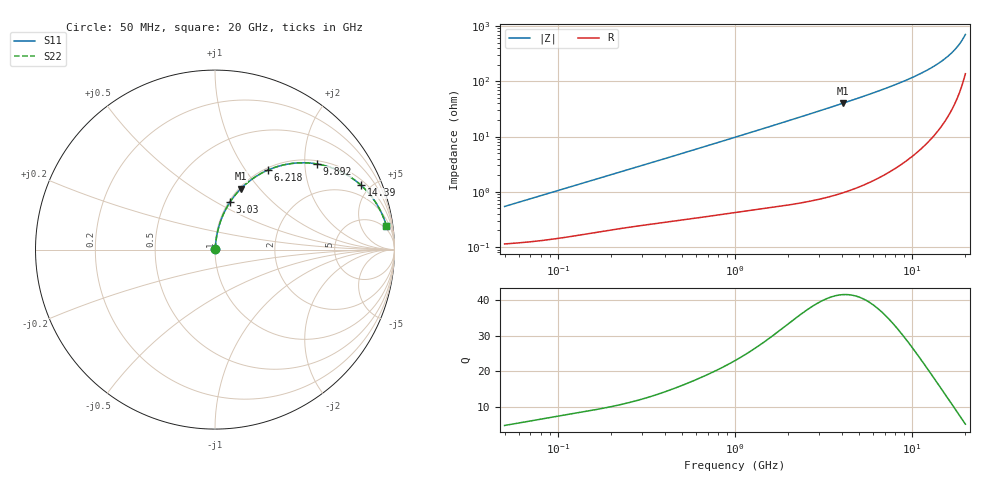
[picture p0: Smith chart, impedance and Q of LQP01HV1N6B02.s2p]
!Murata Part Number: LQP01HV1N6B02
!These Parameters are Measured in Series Mode Connection
!  o--[Z]--o
!Port1  Port2
!  o-------o
!Freq. Start=50[MHz] Stop=20[GHz], 401[Steps]
# Hz S RI R 50
!Freq.(Hz) S11(Real) S11(Imag) S21(Real) S21(Imag) S12(Real) S12(Imag) S22(Real) S22(Imag)
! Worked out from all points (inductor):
!   401 points, 50 MHz to 20 GHz, reference 50 ohm
!   read as one part in series: L = 1.69 nH near 51.52 MHz
!   highest Q = 41.6 at 4.088 GHz (marker M1), where L = 1.56 nH
!   S11 on the Smith chart (normalised r, x): 50 MHz: 1.00, +0.01; 3.03 GHz: 1.01, +0.59; 6.218 GHz: 1.03, +1.27; 9.892 GHz: 1.08, +2.29; 14.39 GHz: 1.28, +4.39; 20 GHz: 4, +14
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5e7  0.00117 0.0053  0.9988 -0.0053  0.9988 -0.0053  0.00117 0.0053
1.364002e8  0.00187 0.0141  0.9981 -0.0141  0.9981 -0.0141  0.00187 0.0141
3.721004e8  0.00406 0.0367  0.9959 -0.0367  0.9959 -0.0367  0.00406 0.0367
6.285508e8  0.00712 0.0608  0.9929 -0.0608  0.9929 -0.0608  0.00712 0.0608
1e9  0.0134 0.0951  0.9866 -0.0951  0.9866 -0.0951  0.0134 0.0951
1.689197e9  0.0307 0.1569  0.9693 -0.1569  0.9693 -0.1569  0.0307 0.1569
2.728004e9  0.0707 0.2436  0.9293 -0.2436  0.9293 -0.2436  0.0707 0.2436
3.029571e9  0.0852 0.2669  0.9148 -0.2669  0.9148 -0.2669  0.0852 0.2669
4.087748e9  0.1449 0.3402  0.8551 -0.3402  0.8551 -0.3402  0.1449 0.3402
5.041459e9  0.208 0.3938  0.792 -0.3938  0.792 -0.3938  0.208 0.3938
6.217679e9  0.2935 0.4425  0.7065 -0.4425  0.7065 -0.4425  0.2935 0.4425
7.442007e9  0.3864 0.4727  0.6136 -0.4727  0.6136 -0.4727  0.3864 0.4727
8.644534e9  0.4767 0.4835  0.5233 -0.4835  0.5233 -0.4835  0.4767 0.4835
9.892087e9  0.5656 0.4775  0.4344 -0.4775  0.4344 -0.4775  0.5656 0.4775
1.201863e10  0.6987 0.4358  0.3013 -0.4358  0.3013 -0.4358  0.6987 0.4358
1.314879e10  0.7582 0.4018  0.2418 -0.4018  0.2418 -0.4018  0.7582 0.4018
1.438523e10  0.8139 0.3584  0.1861 -0.3584  0.1861 -0.3584  0.8139 0.3584
1.573793e10  0.8638 0.3059  0.1362 -0.3059  0.1362 -0.3059  0.8638 0.3059
1.721783e10  0.9061 0.2453  0.0939 -0.2453  0.0939 -0.2453  0.9061 0.2453
1.828096e10  0.9292 0.201  0.0708 -0.201  0.0708 -0.201  0.9292 0.201
1.940974e10  0.9478 0.1541  0.0522 -0.1541  0.0522 -0.1541  0.9478 0.1541
2e10  0.9553 0.1299  0.0447 -0.1299  0.0447 -0.1299  0.9553 0.1299
